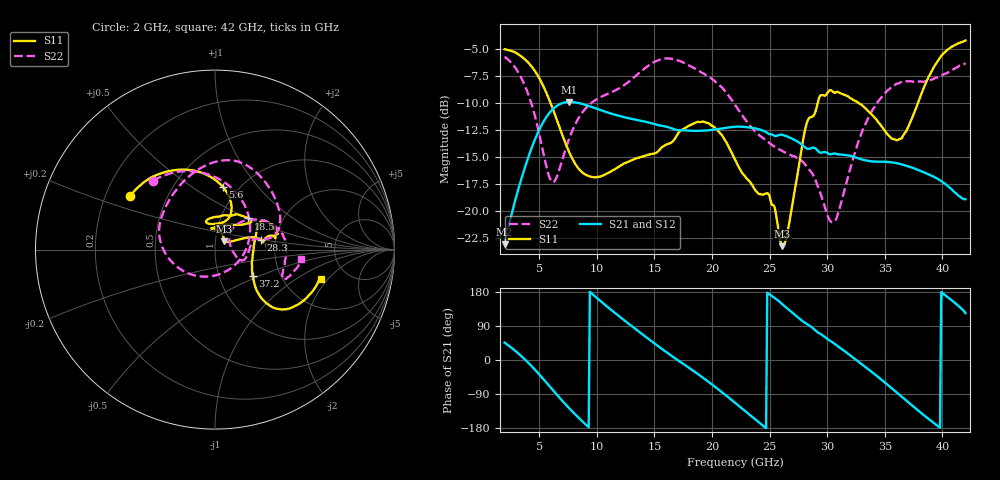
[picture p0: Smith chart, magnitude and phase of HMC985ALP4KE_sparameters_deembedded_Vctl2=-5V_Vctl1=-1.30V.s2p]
!s2p File: Measurements: S11, S21, S12, S22
# GHz S dB R 50.0
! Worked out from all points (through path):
!   401 points, 2 GHz to 42 GHz, reference 50 ohm
!   highest |S21| = -9.93 dB at 7.6 GHz (marker M1); lowest = -23.1 dB at 2 GHz (marker M2)
!   lowest |S11| = -23.3 dB at 26.1 GHz (marker M3), VSWR 1.15, Z = 55.1 + j5.13 ohm
!   |S11| at or under -10 dB: 5.98 GHz to 29.18 GHz (23.2 GHz wide, 132 % of centre); 32.69 GHz to 37.89 GHz (5.2 GHz wide, 14.7 % of centre)
!   |S22| runs from -21.1 to -5.7 dB; largest |S21 - S12| = 0.00036
!   S11 on the Smith chart (normalised r, x): 2 GHz: 0.30, +0.26; 5.6 GHz: 0.84, +0.68; 18.5 GHz: 1.35, +0.50; 28.3 GHz: 1.67, +0.20; 37.2 GHz: 1.45, -0.45; 42 GHz: 3.22, -1.69
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2  -5.05 148.0  -23.11 45.8  -23.12 45.9  -5.75 131.7
3.6  -5.85 121.5  -16.54 6.1  -16.54 6.1  -8.04 87.4
4.7  -7.18 100.6  -13.24 -27.7  -13.24 -27.7  -11.51 45.5
5.6  -9.03 83.1  -11.37 -58.6  -11.38 -58.6  -15.79 -8.2
6.3  -10.90 72.4  -10.48 -83.3  -10.49 -83.3  -17.31 -69.2
7.6  -14.56 66.9  -9.93 -127.2  -9.94 -127.2  -13.33 -147.5
8.7  -16.41 77.9  -10.10 -160.6  -10.11 -160.6  -10.96 -178.0
10.1  -16.87 96.0  -10.59 161.2  -10.60 161.2  -9.61 160.3
12  -15.86 108.0  -11.24 113.9  -11.24 114.0  -8.63 135.5
15.4  -14.42 80.1  -12.10 35.0  -12.10 35.0  -6.05 84.9
18.5  -11.89 43.0  -12.61 -31.1  -12.61 -31.1  -6.83 47.4
22  -15.25 52.9  -12.22 -113.0  -12.23 -113.0  -10.19 11.8
24.9  -18.41 94.9  -12.86 175.4  -12.87 175.5  -13.65 10.5
26.1  -23.27 42.5  -12.97 147.5  -12.98 147.5  -14.47 -2.2
28.3  -11.67 12.3  -14.26 93.9  -14.26 94.0  -15.99 -22.1
28.7  -11.30 8.9  -14.17 85.5  -14.18 85.5  -16.52 -22.1
30.6  -9.06 15.4  -14.70 43.6  -14.70 43.6  -21.02 21.5
33.1  -10.30 31.2  -15.28 -13.4  -15.28 -13.4  -12.49 43.5
35.4  -13.09 8.8  -15.50 -69.2  -15.50 -69.2  -8.75 19.3
37.2  -11.85 -34.8  -15.95 -115.4  -15.95 -115.4  -8.01 -1.2
39.7  -5.97 -41.6  -17.12 -176.4  -17.11 -176.4  -7.60 -23.6
42  -4.24 -15.5  -18.92 123.9  -18.93 123.9  -6.33 -5.9
